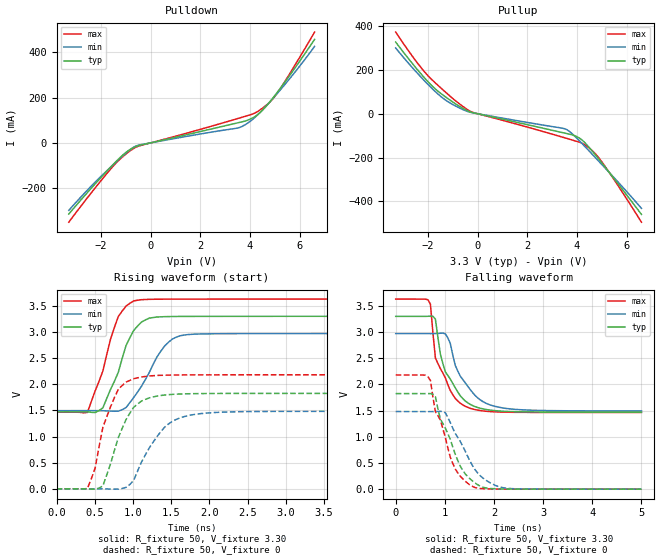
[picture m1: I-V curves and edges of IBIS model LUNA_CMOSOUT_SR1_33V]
[IBIS Ver]   3.2
[Comment Char]   |_char
[File name]   sg8201cga_33v_d.ibs
[File Rev]   1.1
[Date]   2021/10/19 9:35:58
[Source]
[Notes]
[Disclaimer]
This information is for modeling purposes only, and is not guaranteed.
Property of SEIKO EPSON Corp.,
unauthorized reproduction and/or distribution is strictly prohibited.
[Copyright]
Copyright 2021, SEIKO EPSON Corp.
[Component]   2G005_2016
Si_location Pin
Timing_location Pin
[Manufacturer]   SEIKO EPSON Corp.
| 2016 PKG
[Package]
R_pkg   42m   NA   NA
L_pkg   0.49n   NA   NA
C_pkg   0.178p   NA   NA
[Pin] signal_name   model_name
1   OE   NC
2   GND   GND
3   OUT   LUNA_CMOSOUT_SR1_33V
4   VCC   POWER
| Models and submodels in the file (1): LUNA_CMOSOUT_SR1_33V (Output)
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[Model]   LUNA_CMOSOUT_SR1_33V
Model_type Output
Polarity Non-Inverting
Vmeas=1.65
C_comp   2.5p   2.0p   3.0p
[Temperature Range] 25   140   -40
[Voltage Range]   3.30   2.97   3.63
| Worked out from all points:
|   slope of the pulldown table from 0 to 0.495 V, typ, clamps not added: 40.7 ohm
|   slope of the pullup table from 0 to 0.495 V, typ, clamps not added: 40.9 ohm
|   falling waveform, R_fixture 50, V_fixture 3.30: 20-80 % time 422ps typ, 480ps min, 367ps max; typ from 3.3 V to 1.47 V
|   falling waveform, R_fixture 50, V_fixture 0: 20-80 % time 483ps typ, 529ps min, 428ps max; typ from 1.82 V to 0 V
|   rising waveform, R_fixture 50, V_fixture 3.30: 20-80 % time 287ps typ, 355ps min, 271ps max; typ from 1.47 V to 3.3 V
|   rising waveform, R_fixture 50, V_fixture 0: 20-80 % time 284ps typ, 372ps min, 247ps max; typ from 0 V to 1.82 V
[Pullup]
-3.3V     327.2mA    300.4mA    372.8mA
-2.4V     198mA      181.9mA    228.1mA
-1.8V     123.4mA    111.4mA    151.1mA
-1.2V     69.34mA    55.35mA    89.15mA
-400mV    13.37mA    10.29mA    18.3mA
-100mV    2.444mA    2.017mA    2.954mA
3.5V      -88.24mA   -68.33mA   -109.6mA
4V        -104.9mA   -112.1mA   -126.5mA
4.4V      -141.8mA   -159.1mA   -148.3mA
4.7V      -181.9mA   -195.2mA   -177.7mA
5V        -224.3mA   -231.5mA   -219mA
6.6V      -459.6mA   -432mA     -495.2mA
[Pulldown]
-3.3V     -314.6mA   -298.3mA   -350.7mA
-2.5V     -213.4mA   -203.1mA   -235.6mA
-1.6V     -105.8mA   -105.8mA   -113.9mA
-1.1V     -51.38mA   -55.23mA   -58.89mA
-700mV    -21.32mA   -20.13mA   -25.77mA
-300mV    -7.362mA   -6.024mA   -8.697mA
3.6V      90.83mA    68.7mA     110.4mA
4.2V      116.2mA    112.7mA    131.8mA
4.6V      155.8mA    156.7mA    161.5mA
4.9V      195.1mA    193.1mA    191.9mA
5.2V      238.1mA    231.3mA    236.4mA
6.6V      457.2mA    426.1mA    489.4mA
[Falling Waveform]
R_fixture=50
V_fixture=3.30
V_fixture_min=2.97
V_fixture_max=3.63
0s        3.3V       2.97V      3.63V
656.6ps   3.301V     2.97V      3.617V
707.1ps   3.302V     2.97V      3.531V
808.1ps   3.246V     2.97V      2.504V
909.1ps   2.581V     2.977V     2.302V
1.01ns    2.241V     2.966V     2.125V
1.212ns   1.936V     2.365V     1.732V
1.414ns   1.685V     2.032V     1.583V
2.172ns   1.489V     1.552V     1.471V
5ns       1.472V     1.495V     1.465V
[Falling Waveform]
R_fixture=50
V_fixture=0
V_fixture_min=0
V_fixture_max=0
0s        1.825V     1.482V     2.181V
656.6ps   1.826V     1.482V     2.146V
707.1ps   1.825V     1.482V     2.075V
808.1ps   1.765V     1.482V     1.478V
909.1ps   1.338V     1.487V     1.319V
1.01ns    1.164V     1.46V      983.9mV
1.162ns   805mV      1.163V     492.5mV
1.566ns   154.4mV    445.1mV    51.2mV
2.222ns   3.705mV    22.01mV    1.756mV
5ns       372.4uV    613.3uV    233.5uV
[Rising Waveform]
R_fixture=50
V_fixture=3.30
V_fixture_min=2.97
V_fixture_max=3.63
0s        1.472V     1.495V     1.465V
404ps     1.471V     1.495V     1.461V
606.1ps   1.549V     1.494V     2.254V
808.1ps   2.23V      1.485V     3.296V
909.1ps   2.74V      1.554V     3.496V
1.01ns    3.031V     1.747V     3.595V
1.212ns   3.265V     2.223V     3.625V
1.414ns   3.293V     2.733V     3.628V
1.616ns   3.297V     2.928V     3.629V
5ns       3.3V       2.97V      3.63V
[Rising Waveform]
R_fixture=50
V_fixture=0
V_fixture_min=0
V_fixture_max=0
0s        0V         549.3nV    0V
404ps     -585.7uV   220.8uV    7.174mV
505.1ps   -7.172mV   390.2uV    396.2mV
606.1ps   55.62mV    -725.6uV   1.177V
808.1ps   979.8mV    -6.508mV   1.903V
1.01ns    1.562V     164.8mV    2.106V
1.162ns   1.71V      649.8mV    2.149V
1.364ns   1.785V     1.093V     2.171V
1.717ns   1.818V     1.399V     2.179V
5ns       1.825V     1.482V     2.181V
[Ramp]
R_load=50
dV/dt_r   1.095E+0/2.832E-10   8.892E-1/3.716E-10   1.308E+0/2.472E-10
dV/dt_f   1.097E+0/4.212E-10   8.852E-1/4.801E-10   1.299E+0/3.647E-10
|[End   LUNA_CMOSOUT_SR1_33V
